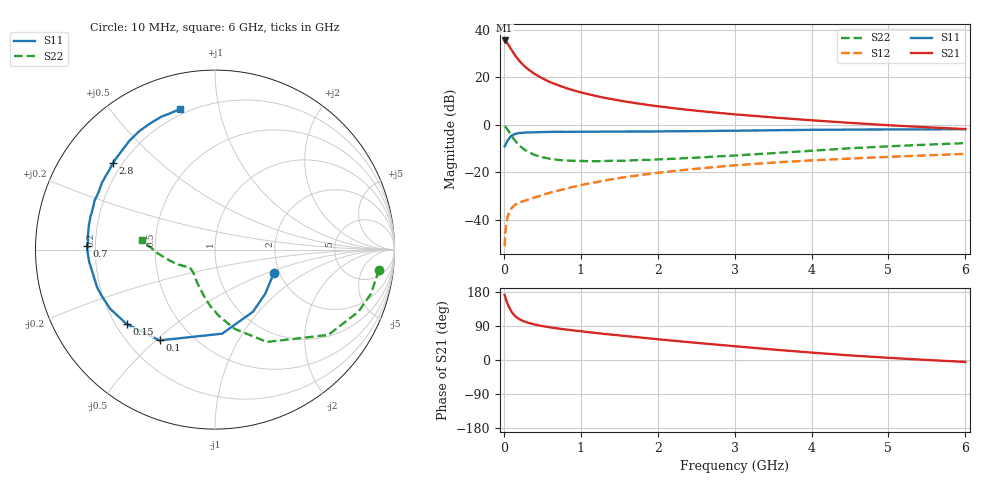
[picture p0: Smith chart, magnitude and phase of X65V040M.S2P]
! SIEMENS Small Signal Semiconductors
! BFP193W
! Si NPN RF Bipolar Junction Transistor in SOT343
! VCE = 5 V  IC = 40 mA
! Common Emitter S-Parameters:  April 1994
# GHz  S  MA  R  50
!  f  S11  S21  S12  S22
! GHz  MAG  ANG  MAG  ANG  MAG  ANG  MAG  ANG
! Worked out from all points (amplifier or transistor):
!   40 points, 10 MHz to 6 GHz, reference 50 ohm
!   highest |S21| = 35.5 dB at 10 MHz (marker M1)
!   |S21| within 3 dB of that: start of sweep to 81.3 MHz
!   unconditionally stable (mu >= 1): 732.4 MHz to 3.98 GHz
!   at 200 MHz: K = 0.51, MSG = 29.9 dB, |S12| = -32.8 dB
!   at 1.5 GHz: K = 1.12, MAG = 14.2 dB, |S12| = -22.4 dB
!   at 6 GHz: K = 0.94, MSG = 5.2 dB, |S12| = -12.2 dB
!   S11 on the Smith chart (normalised r, x): 10 MHz: 1.88, -0.55; 100 MHz: 0.33, -0.51; 150 MHz: 0.24, -0.35; 700 MHz: 0.17, +0.01; 2.8 GHz: 0.16, +0.36; 6 GHz: 0.17, +0.77
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0.01  0.3531 -21.3  59.37 171.7  0.0028 82.9  0.9212 -7.0
0.02  0.3726 -41.3  58.23 165.4  0.0055 74.0  0.9027 -15.9
0.03  0.4056 -58.5  56.34 158.8  0.008 73.3  0.8708 -23.4
0.05  0.4701 -85.1  50.87 146.9  0.012 63.9  0.79 -37.0
0.1  0.5926 -121.4  37.5 126.9  0.0178 50.0  0.5901 -60.7
0.15  0.6437 -139.9  28.23 115.0  0.0211 44.8  0.454 -76.2
0.2  0.6707 -150.5  22.2 107.9  0.0229 44.2  0.3694 -86.7
0.25  0.6813 -157.5  18.29 102.9  0.0246 44.6  0.3164 -94.7
0.3  0.6896 -162.2  15.38 99.2  0.0262 45.1  0.2761 -101.4
0.4  0.6941 -169.3  11.73 93.7  0.0296 48.1  0.2323 -111.2
0.5  0.7038 -174.2  9.476 89.5  0.0334 51.3  0.208 -118.8
0.6  0.7092 -178.2  7.922 86.2  0.0372 53.3  0.1927 -124.7
0.7  0.7134 178.5  6.856 83.3  0.041 55.4  0.1828 -129.1
0.9  0.7127 173.4  5.339 78.1  0.0495 58.0  0.1749 -135.4
1.1  0.7153 169.2  4.394 73.5  0.0582 59.2  0.1714 -139.8
1.6  0.7211 159.5  3.05 62.8  0.0802 59.9  0.1762 -145.5
2.2  0.7315 149.4  2.241 51.0  0.1063 57.4  0.1927 -151.6
2.8  0.746 139.8  1.776 40.0  0.1317 53.7  0.2175 -156.9
3.2  0.7559 133.8  1.563 32.9  0.1478 50.9  0.2367 -161.5
4.5  0.7909 116.9  1.098 12.1  0.195 41.4  0.3206 -176.4
5.5  0.7994 108.3  0.886 0.1  0.2279 34.9  0.3825 175.5
6  0.8073 103.9  0.814 -5.1  0.2451 32.0  0.4119 172.5
